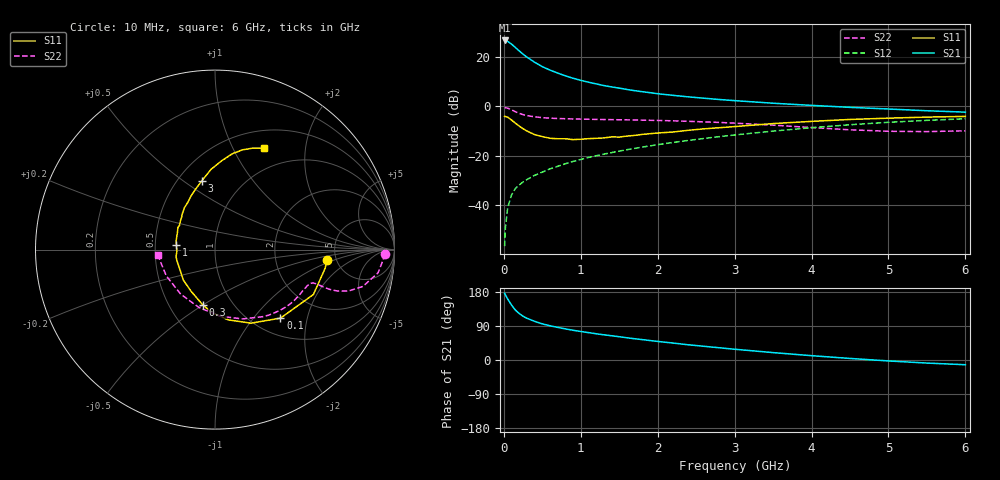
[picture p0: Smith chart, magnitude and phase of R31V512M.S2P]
! SIEMENS Small Signal Semiconductors
! BFR181
! Si NPN RF Bipolar Junction Transistor in SOT23
! VCE = 1.5 V  IC = 12 mA
! Common Emitter S-Parameters:  May  1996
# GHz  S  MA  R  50
!  f  S11  S21  S12  S22
! GHz  MAG  ANG  MAG  ANG  MAG  ANG  MAG  ANG
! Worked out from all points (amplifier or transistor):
!   36 points, 10 MHz to 6 GHz, reference 50 ohm
!   highest |S21| = 26.6 dB at 10 MHz (marker M1)
!   |S21| within 3 dB of that: start of sweep to 155.9 MHz
!   unconditionally stable (mu >= 1): 417.7 MHz to 3.162 GHz
!   at 250 MHz: K = 0.79, MSG = 25.8 dB, |S12| = -30.5 dB
!   at 1.4 GHz: K = 1.19, MAG = 10.6 dB, |S12| = -18.7 dB
!   at 6 GHz: K = 0.95, MSG = 1.3 dB, |S12| = -5.0 dB
!   S11 on the Smith chart (normalised r, x): 10 MHz: 4.20, -0.82; 100 MHz: 1.31, -1.39; 300 MHz: 0.73, -0.50; 1 GHz: 0.65, +0.03; 3 GHz: 0.65, +0.59; 6 GHz: 0.72, +1.33
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0.01  0.6275 -5.4  21.34 176.0  0.0015 91.5  0.9456 -1.5
0.02  0.6219 -9.8  21.05 172.0  0.0035 78.4  0.939 -3.4
0.05  0.6027 -24.5  20.43 161.0  0.009 78.2  0.9177 -8.1
0.1  0.5281 -46.3  18.02 144.9  0.0162 71.9  0.8489 -14.0
0.15  0.4565 -63.9  15.4 131.8  0.0219 66.6  0.7772 -17.3
0.2  0.398 -79.5  13.14 122.7  0.0259 65.7  0.7208 -18.7
0.25  0.3526 -92.2  11.25 115.4  0.0297 64.0  0.6787 -19.1
0.3  0.3171 -102.1  9.849 110.1  0.0332 64.9  0.649 -19.1
0.4  0.2676 -119.9  7.757 102.0  0.0404 65.6  0.6135 -18.8
0.5  0.2449 -136.1  6.312 95.3  0.0468 67.2  0.5895 -18.7
0.6  0.2261 -148.6  5.384 90.3  0.0546 68.8  0.5759 -18.8
0.7  0.2212 -159.6  4.687 86.0  0.0614 69.7  0.5666 -19.3
0.8  0.2211 -169.4  4.129 82.1  0.0693 69.9  0.5609 -19.8
1  0.216 173.7  3.344 75.3  0.0845 70.8  0.5512 -21.6
1.1  0.2223 166.6  3.065 72.3  0.0927 71.1  0.5478 -22.8
1.6  0.2503 140.4  2.187 58.7  0.133 69.9  0.5324 -29.1
2.2  0.3028 120.2  1.663 44.7  0.1862 66.7  0.5088 -38.8
3  0.3898 100.9  1.302 28.4  0.2636 60.1  0.4577 -54.8
3.5  0.4479 92.8  1.153 19.5  0.3156 54.9  0.416 -68.2
4.5  0.5425 79.8  0.952 4.1  0.4241 42.2  0.3351 -105.3
5.5  0.605 69.3  0.813 -8.1  0.5204 27.6  0.3083 -151.6
6  0.6254 64.4  0.762 -12.5  0.5603 19.9  0.3203 -174.5
